PROGRAM MAIN
VAR
   TxPDO_toggle_prim   AT%I*    :  BOOL; // Sets Device 1 Sync-Master
   TxPDO_toggle_sec    AT%I*    :  BOOL; // Sets Device 3 Sync-Master
// Sync Master for Devices needed to set EL6695 in OP mode on prim. and sec. side
END_VAR

END_PROGRAM
